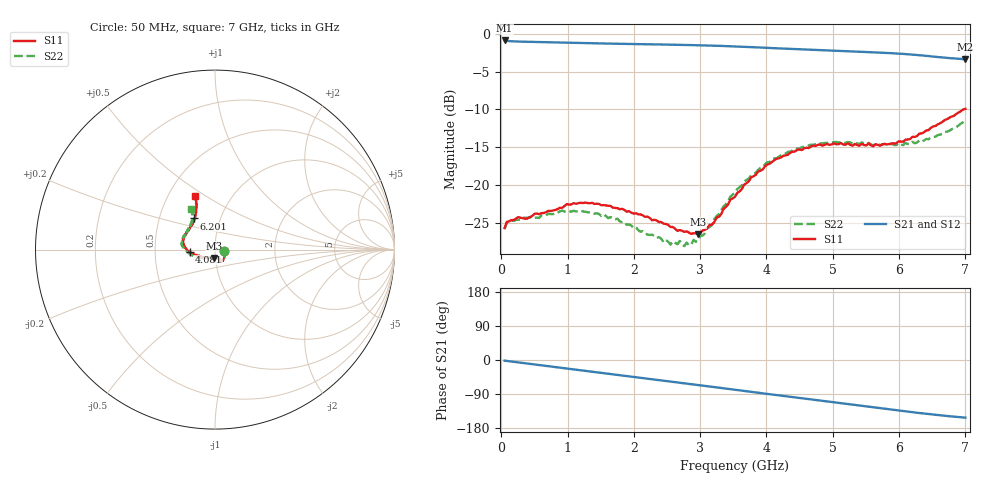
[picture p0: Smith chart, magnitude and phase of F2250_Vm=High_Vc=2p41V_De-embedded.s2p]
! Integrated Device Technology
! Corporate Headquarters
! 6024 Silver Creek Valley Road
! San Jose, CA 95138  USA
! Phone:  1-408-284-8200
! Toll Free:  1-800-223-1366
! Webpage:  http://www.idt.com/
! Timing and RF Division
! 515 Groton Road, Suite 102
! Westford, MA 01886-6024
! Device:  F2250
! Description: Voltage Variable RF Attenuator
! Frequency:  50.0 -  6000.00 MHz
! Package:  3x3 mm Thin QFN Plastic Package: 16 pin
! Ports:  2 RF, 3 DC
!  Pin  1  = GND
!  Pin  2  = NC
!  Pin  3  = RF1  = Port 1
!  Pin  4  = NC
!  Pin  5  = GND
!  Pin  6  = GND
!  Pin  7  = GND
!  Pin  8  = GND
!  Pin  9  = NC
!  Pin 10  = RF2  = Port 2
!  Pin 11  = NC
!  Pin 12  = GND
!  Pin 13  = GND
!  Pin 14  = VCNTRL
!  Pin 15  = VDD
!  Pin 16  = VMODE
! Vcntrl:  2.410 Volts
! Vmode:  +3.300 Volts
! Vdd:  +3.30  Volts
! Current:  1.314 mA
! Data:  The device was measured on a the F2250 evaluation board which has
!  individual transmission lines to the RF pins.  Data was collected
!  using a calibrated network analyzer.  The evaluation board was
!  de-embedded using a TRL calibration technique.
!  The reference plane is the edge of the package pin.
! Misc:  SN 10
!  Action Tracker AT0258
! Date Measured:  2014-11-26
! Date:  2015-10-15  MJV
! Note:
!  Integrated Device Technology supplies this data as a sample of measured
!  data at the package pin for this product.  Your particular data for this
!  product may vary.
!  Data was taken at 25 degrees C.
!  Integrated Device Technology reserves the right to change this data at anytime.
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# GHz S dB R 50
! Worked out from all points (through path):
!   201 points, 50 MHz to 7 GHz, reference 50 ohm
!   highest |S21| = -0.89 dB at 50 MHz (marker M1); lowest = -3.4 dB at 7 GHz (marker M2)
!   group delay of S21, straight-line fit = 61.2 ps
!   lowest |S11| = -26.5 dB at 2.969 GHz (marker M3), VSWR 1.10, Z = 49.2 - j4.62 ohm
!   |S11| at or under -10 dB: start of sweep to 6.968 GHz
!   |S22| runs from -28.0 to -11.6 dB; largest |S21 - S12| = 0.0019
!   S11 on the Smith chart (normalised r, x): 50 MHz: 1.11, -0.02; 4.081 GHz: 0.75, -0.02; 6.201 GHz: 0.75, +0.27; 7 GHz: 0.68, +0.45
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0.05  -25.65 -10.6  -0.89 -1.8  -0.89 -1.8  -25.81 -10.9
0.1195  -24.75 -10.2  -0.99 -3.2  -0.98 -3.2  -24.68 -8.9
0.57125  -23.83 -31.3  -1.10 -13.3  -1.10 -13.3  -24.33 -31.4
0.91875  -22.99 -50.1  -1.17 -21.0  -1.17 -21.1  -23.35 -51.0
1.2315  -22.36 -57.9  -1.24 -27.9  -1.24 -27.9  -23.46 -61.5
1.75275  -23.03 -64.8  -1.33 -39.1  -1.33 -39.1  -24.42 -67.8
2.37825  -24.86 -64.5  -1.42 -52.8  -1.42 -52.8  -26.85 -66.8
2.552  -25.51 -69.4  -1.45 -56.7  -1.45 -56.7  -27.84 -73.1
2.691  -25.92 -77.5  -1.47 -59.8  -1.47 -59.8  -27.36 -81.0
2.7605  -26.16 -79.7  -1.48 -61.3  -1.49 -61.3  -28.05 -85.3
2.969  -26.49 -97.7  -1.52 -66.0  -1.52 -66.0  -27.27 -105.0
3.1775  -25.21 -120.8  -1.57 -70.7  -1.57 -70.7  -25.24 -126.8
3.525  -21.54 -152.7  -1.68 -78.5  -1.68 -78.6  -20.97 -148.8
3.76825  -18.97 -164.8  -1.77 -84.0  -1.77 -84.1  -18.69 -159.7
4.081  -16.95 -175.7  -1.90 -91.0  -1.90 -91.0  -16.72 -171.5
4.4285  -15.54 176.0  -2.03 -98.6  -2.04 -98.7  -15.20 178.6
4.7065  -14.76 169.1  -2.13 -104.8  -2.13 -104.8  -14.69 172.9
5.054  -14.61 160.9  -2.26 -112.5  -2.26 -112.5  -14.29 165.9
5.85325  -14.57 135.1  -2.56 -130.0  -2.56 -130.1  -14.69 147.2
6.20075  -13.61 123.6  -2.77 -137.7  -2.77 -137.8  -14.27 138.2
6.54825  -12.18 115.6  -3.04 -144.7  -3.04 -144.9  -13.60 126.8
7  -9.91 110.8  -3.37 -152.1  -3.38 -152.2  -11.56 120.6
